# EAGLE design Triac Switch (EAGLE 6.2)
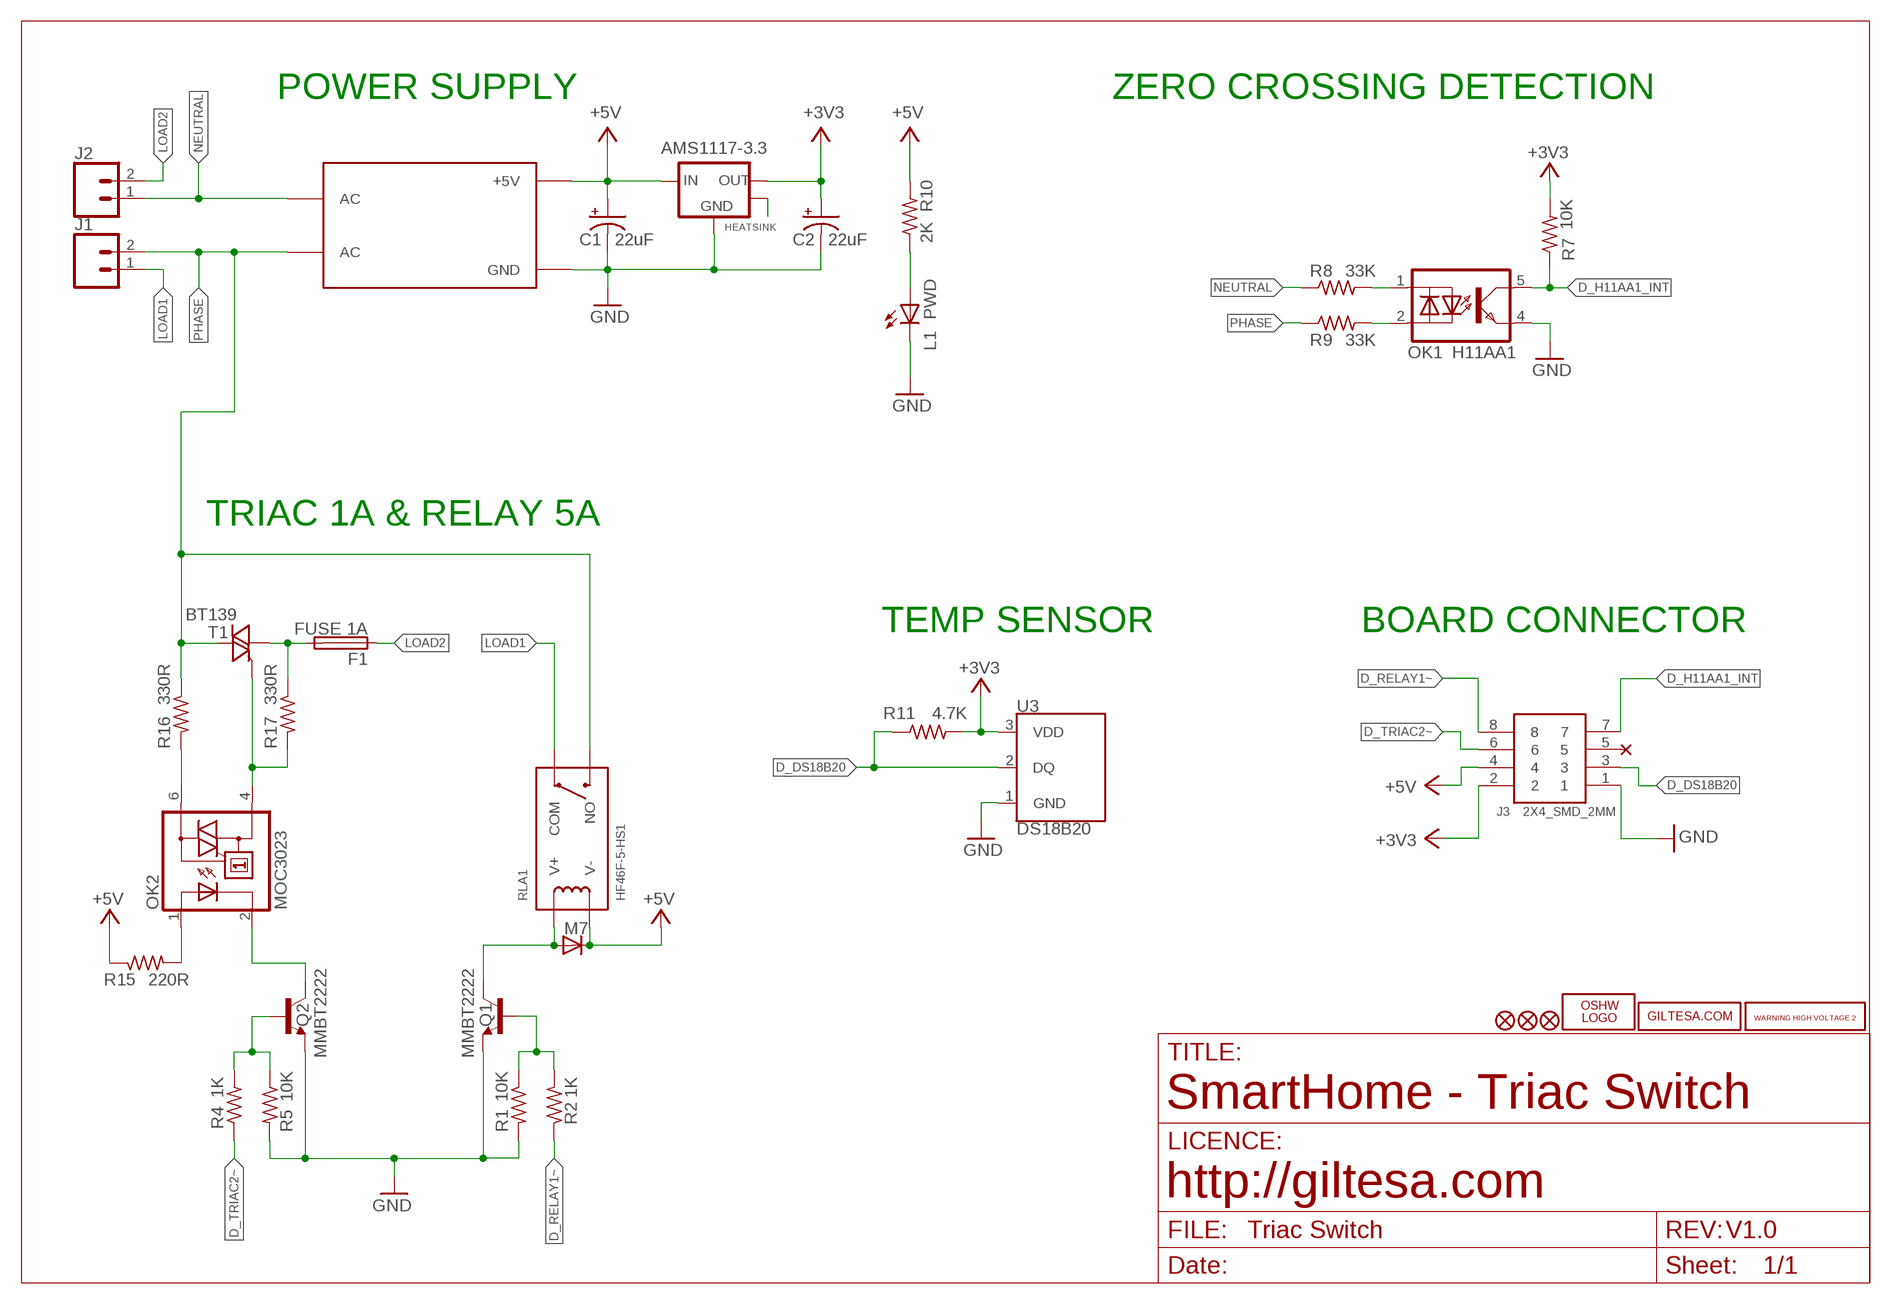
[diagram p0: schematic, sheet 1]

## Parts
AMS1117-3.3  AMS1117SOT89_2  [SOT89_2]
C1  22uF  CAP_POL3528  [EIA3528]
C2  22uF  CAP_POL3528  [EIA3528]
D1  M7  DIODE-SMB  [SMB]
F1  FUSE 1A  FUSETE5  [TE5]
J1  TERMINAL_5MM_2P_90º  [TERMINAL_5MM_2P_90º]
J2  TERMINAL_5MM_2P_90º  [TERMINAL_5MM_2P_90º]
J3  2X4_SMD_2MM  2X4_SMD_2.0MM  [2X4_SMD_2.0MM]
L1  PWD  LEDCHIP-LED0805  [CHIP-LED0805]
LOGO1  OSHW_LOGO_FILLX0150-NT  [OSHW_FILLX150_NOTEXT]
OK1  H11AA1  [H11AA1]
OK2  MOC3023  MOC3021MSMD  [DIL6-SMD]
Q1  MMBT2222  TRANSISTOR_NPNSOT23  [SOT23]
Q2  MMBT2222  TRANSISTOR_NPNSOT23  [SOT23]
R1  10K  R0603  [R0603]
R2  1K  R0603  [R0603]
R4  1K  R0603  [R0603]
R5  10K  R0603  [R0603]
R7  10K  R0603  [R0603]
R8  33K  R1206  [R1206]
R9  33K  R1206  [R1206]
R10  2K  R0603  [R0603]
R11  4.7K  R0603  [R0603]
R15  220R  R0603  [R0603]
R16  330R  R1206  [R1206]
R17  330R  R1206  [R1206]
RLA1  HF46F-5-HS1  RELAY_HF46F-5-HS1  [RELAY_HF46F-5-HS1]
T1  BT139  BT138-V  [TO220BV]
U3  DS18B20  [DS18B20]
U$1  HILINK_HLK-PM01_5V  [HILINK_HLK-PM01_5V]
U$4  WARNING_HIGH_VOLTAGE_2  [WARNING_HIGH_VOLTAGE_2]
U$5  GILTESA.COM_MASK  [GILTESA.COM_MASK]
U$6  FIDUCIAL1X2  [FIDUCIAL-1X2]
U$7  FIDUCIAL1X2  [FIDUCIAL-1X2]
U$14  FIDUCIAL1X2  [FIDUCIAL-1X2]

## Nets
+3V3: AMS1117-3.3.2(OUT) C2.A(+) J3.2 R7.2 R11.2 U3.3(VDD)
+5V: AMS1117-3.3.3(IN) C1.A(+) D1.C J3.4 R10.2 R15.1 RLA1.V- U$1.+5V
D_DS18B20: J3.3 R11.1 U3.2(DQ)
D_H11AA1_INT: J3.7 OK1.5 R7.1
D_RELAY1~: J3.8 R2.1
D_TRIAC2~: J3.6 R4.1
GND: AMS1117-3.3.1(GND) C1.C(-) C2.C(-) J3.1 L1.C OK1.4 Q1.2(E) Q2.2(E) R1.2 R5.2 U3.1(GND) U$1.GND
HEATSINK: AMS1117-3.3.4(NC)
LOAD1: J1.1 RLA1.COM
LOAD2: F1.1 J2.2
N$1: F1.2 R17.1 T1.T1(A1)
N$2: Q1.1(B) R1.1 R2.2
N$3: D1.A Q1.3(C) RLA1.V+
N$6: OK1.1 R8.2
N$7: OK1.2 R9.2
N$8: L1.A R10.1
N$10: OK2.1(A) R15.2
N$12: OK2.6(A2) R16.2
N$13: OK2.4(A1) R17.2 T1.G
N$46: Q2.1(B) R4.2 R5.1
N$47: OK2.2(C) Q2.3(C)
NEUTRAL: J2.1 R8.1 U$1.AC@2(AC)
PHASE: J1.2 R9.1 R16.1 RLA1.NO T1.T2(A2) U$1.AC@1(AC)
Unconnected: J3.5

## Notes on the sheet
- POWER SUPPLY | ZERO CROSSING DETECTION
- TRIAC 1A & RELAY 5A
- TEMP SENSOR | BOARD CONNECTOR
- SmartHome - Triac Switch
- http://giltesa.com
- V1.0

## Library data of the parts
AMS1117-3.3 = ,giltesa:AMS1117
C1 C2 = SparkFun:CAP_POL: Capacitor Polarized
D1 = diode:DIODE-: DIODE
F1 = fuse:FUSE: Fuse; OC_FARNELL: unknown; OC_NEWARK: unknown
J1 J2 = ,giltesa:TERMINAL_5MM_2P_90º
J3 = ,giltesa:2X4_SMD_2.0MM
L1 = led:LED: LED
LOGO1 = ohw-logo:OSHW_LOGO_FILL
OK1 = ,giltesa:H11AA1
OK2 = optocoupler:MOC30*M: RANDOM-PHASE OPTOISOLATORS TRIAC DRIVER OUTPUT Source: http://www.fairchildsemi.com MOC3020-M.pdf
Q1 Q2 = SparkFun:TRANSISTOR_NPN: Transistor NPN BJT configuration in SOT23 package. MMBT2222 is the common NPN we use. Double check BCE configuration again layout.
R1 R2 R4 R5 R7 R10 R11 R15 = ,giltesa:R0603
R8 R9 R16 R17 = ,giltesa:R1206
RLA1 = ,giltesa:RELAY_HF46F-5-HS1
T1 = triac:BT138: TRIAC Source: http://www.semiconductors.philips.com BT138_SERIES_2.pdf
U3 = ,giltesa:DS18B20
U$1 = ,giltesa:HILINK_HLK-PM01_5V
U$4 = ,giltesa_logos:WARNING_HIGH_VOLTAGE_2
U$5 = ,giltesa_logos:GILTESA.COM_MASK
U$6 U$7 U$14 = SparkFun:FIDUCIAL: Fiducial Alignment Points

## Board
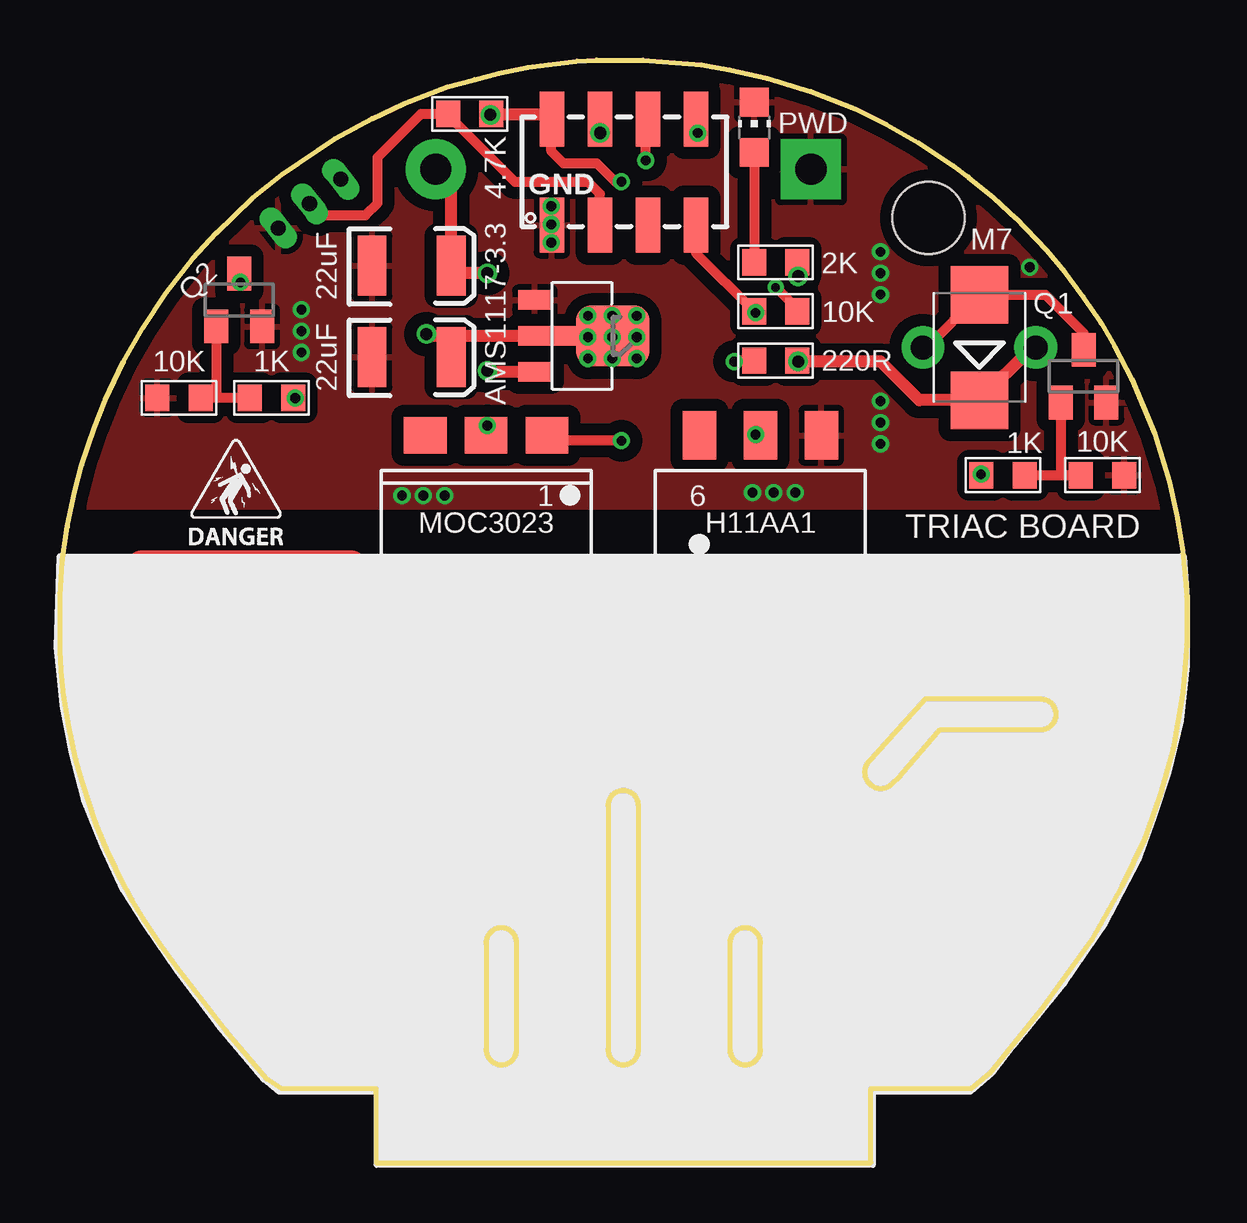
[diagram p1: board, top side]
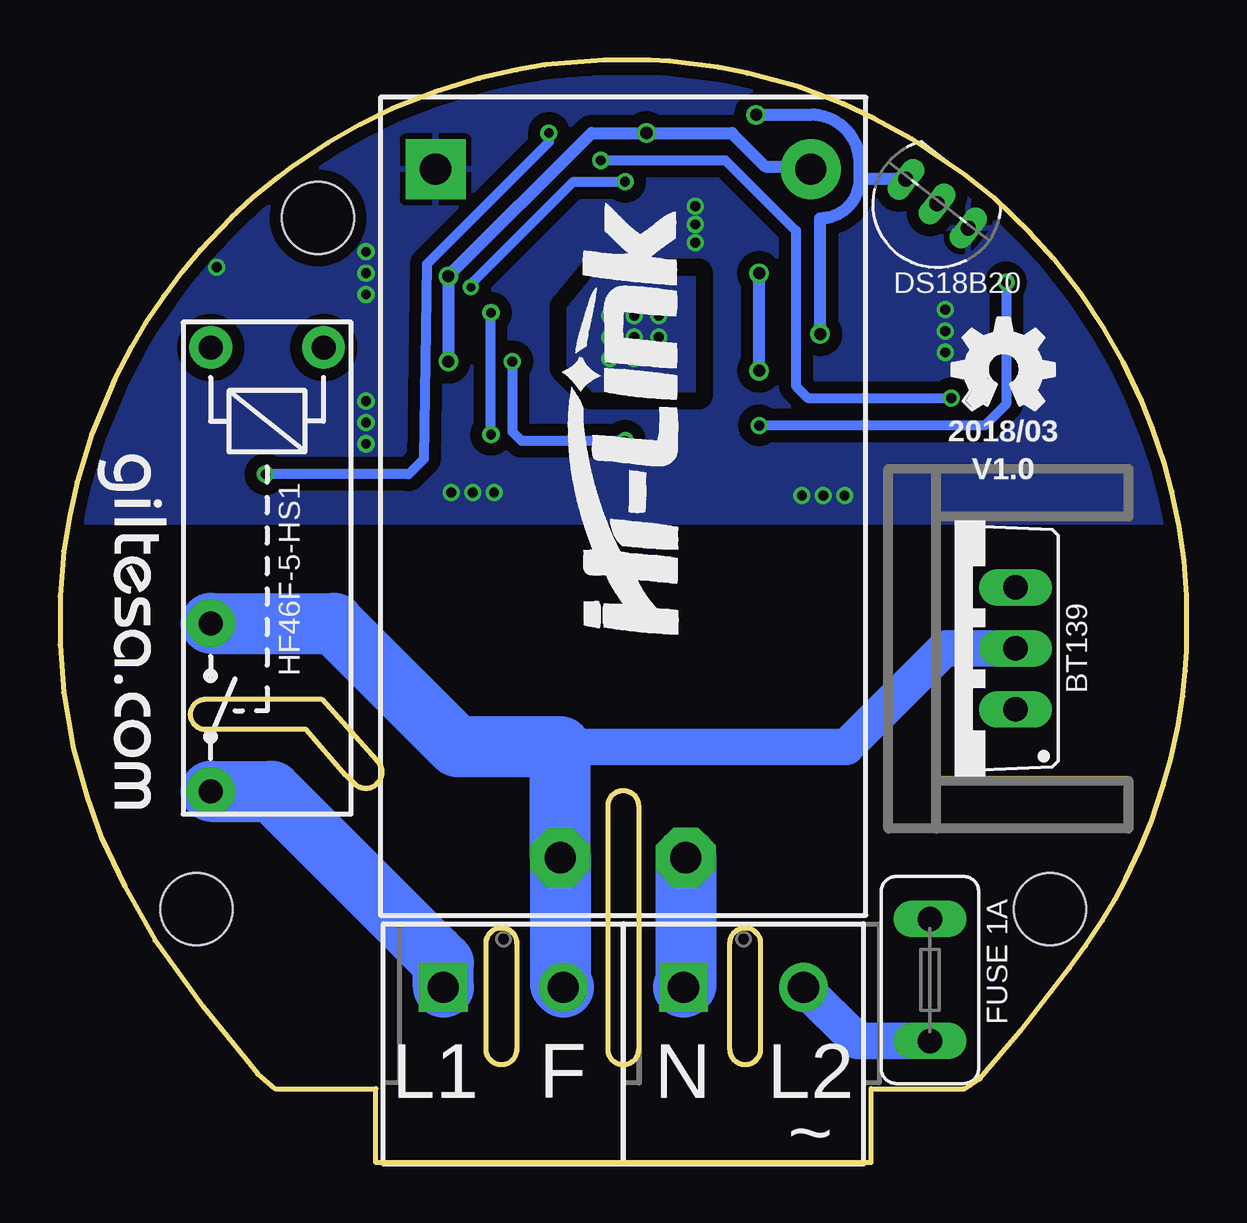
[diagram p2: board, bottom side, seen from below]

Size 46.94 x 45.97 mm. Coordinates in mm from the lower left corner, seen from the top.
Outline: 96 segments
Copper layers (1*16): Top 0.035mm / dielectric 1.6mm / Bottom 0.035mm
Design rules: minimum track width 6mil, minimum drill 12mil, track to track 6mil, track to pad 6mil, pad to pad 6mil, via to via 8mil, smd to smd 0mil, copper to edge 20mil, drill to drill 10mil, minimum pad ring 6mil, minimum via ring 6mil, stop-mask expansion 0mil, vias tented up to drill 100mil, thermal gap 10mil
Holes 3 mm at 5.69,10.57 41.25,10.57 36.19,39.38
bRestrict: 6 lines

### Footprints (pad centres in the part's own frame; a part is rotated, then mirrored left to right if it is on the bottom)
SOT89_2 = smd 0.8 x 1.4: 1 -1.499,-1.981; 3 1.499,-1.981 | smd 0.8 x 2.54: 2 0,-1.409 | smd 2.54 x 3.048: 4 0,1.27
EIA3528 = smd 1.2 x 2.5: A 1.65,0; C -1.65,0
SMB = smd 2.4 x 2.4: A 2.2,0; C -2.2,0
TE5 = drill 1.016 long: 1 -2.54,0; 2 2.54,0
TERMINAL_5MM_2P_90º = drill 1.3 pad 2.032 square: 1 0.004,0 | drill 1.3 pad 2.032: 2 5.004,0
2X4_SMD_2.0MM = smd 2.286 x 1.016: 1 -2.213,2.976; 2 2.212,2.976; 3 -2.213,0.976; 4 2.212,0.976; 5 -2.213,-1.024; 6 2.212,-1.024; 7 -2.213,-3.024; 8 2.212,-3.024
CHIP-LED0805 = smd 1.2 x 1.2: A 0,-1.05; C 0,1.05
H11AA1 = smd 1.397 x 2.032: 1 -2.54,-4.645; 2 0,-4.645; 3 2.54,-4.645; 4 2.54,4.645; 5 0,4.645; 6 -2.54,4.645
DIL6-SMD = smd 1.78 x 1.52: 1 -2.54,-4.645; 2 0,-4.645; 3 2.54,-4.645; 4 2.54,4.645; 5 0,4.645; 6 -2.54,4.645
SOT23 = smd 1 x 1.4: 1 -0.95,-1.1; 2 0.95,-1.1; 3 0,1.1
R0603 = smd 1 x 1.1: 1 -0.901,0.013; 2 0.901,0.013
R1206 = smd 1.6 x 1.8: 1 -1.387,-0.013; 2 1.362,-0.013
RELAY_HF46F-5-HS1 = drill 1 pad 2.032: COM 9.3,-2.35; NO 2.3,-2.35 | drill 1 pad 1.778: V+ -9.2,2.35; V- -9.2,-2.35
TO220BV = drill 1.016 long: G 2.54,-2.54; T1 -2.54,-2.54; T2 0,-2.54
DS18B20 = drill 0.635 pad 0.864 long: 1 -1.651,0; 2 0,0; 3 1.651,0
HILINK_HLK-PM01_5V = drill 1.3 pad 2.5: +5V 31.109,2.3 | drill 1.3 pad 2.5 octagon: AC@1 2.409,12.73; AC@2 2.409,7.5 | drill 1.3 pad 2.5 square: GND 31.109,17.93
FIDUCIAL-1X2 = smd 1 x 1: 1 0,0

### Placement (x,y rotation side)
AMS1117-3.3  21.76,34.46 270 top
C1  14.65,37.38 0 top
C2  14.65,33.57 0 top
D1  38.3,33.98 90 top
F1  10.69,7.62 90 bottom
J1  30.97,7.31 0 bottom
J2  20.97,7.31 0 bottom
J3  23.47,41.29 90 top
L1  28.93,43.16 0 top
LOGO1  9.75,31.39 0 bottom
OK1  29.18,25.67 0 top
OK2  17.75,25.67 180 top
Q1  42.65,32.78 0 top
Q2  7.47,35.96 0 top
R1  43.44,28.65 0 top
R2  39.29,28.65 0 top
R4  8.81,31.89 180 top
R5  4.96,31.89 180 top
R7  29.82,35.48 0 top
R8  24.92,17.39 0 top
R9  30.58,16 90 top
R10  29.82,37.51 0 top
R11  17.07,43.7 0 top
R15  29.82,33.45 180 top
R16  16.66,17.39 0 top
R17  2.44,21.44 90 top
RLA1  38.3,24.78 270 bottom
T1  9.66,21.44 90 bottom
U3  10.4,39.98 142 bottom
U$1  13.36,10.3 90 bottom
U$2  [ELECTROCUTION_SMALL]  5.14,25.63 0 top
U$4  43.03,15.51 0 top
U$5  45.44,29.61 270 bottom
U$6  32.42,1.37 90 top
U$7  23.47,24.66 90 top
U$14  14.54,1.37 90 top

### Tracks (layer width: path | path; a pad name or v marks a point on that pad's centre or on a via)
+3V3  (via drill 0.36, 0.41, 0.51)
  Top 0.406: R7.2 30.72,35.59 v29.82,36.5 | v23.39,40.89 23.14,40.89 22.38,41.65 20.98,41.65 20.47,42.16 20.47,43.48 J3.2
  Top 0.508: AMS1117-3.3.2 16.46,34.46 | 16.46,34.46 16.28,34.29 16.28,33.6 C2.A | 16.46,34.46 15.34,34.46 v15.27,34.54 | J3.2 20.28,43.71 R11.2 17.96,43.71 v17.93,43.68
  Bottom 0.406: v23.39,40.89 25.55,40.89 29.82,36.62 v29.82,36.5
  Bottom 0.508: v15.27,34.54 15.27,39.37 arc-90 13.61,41.02 | v17.93,43.68 15.65,43.68 arc90 13.61,41.65 13.61,41.02 | U3.3 13.59,40.99 arc90 13.61,41.02
+5V  (via drill 0.51)
  Top 0.508: RLA1.V- 40.51,33.98 D1.C 35.81,31.78 34.19,33.4 v30.76,33.4 R15.1 30.76,33.47 v30.76,33.4 | U$1.+5V 16.3,40.77 C1.A 16.61,37.08 v17.81,37.08 | J3.4 22.49,43.06 v22.5,42.92 | 30.82,37.52 R10.2 30.76,37.49 v30.76,36.95 | AMS1117-3.3.3 17.86,32.96 v17.81,33.02
  Bottom 0.508: v17.81,33.02 v17.81,37.08 | 15.66,41.38 U$1.+5V 15.77,41.52 17.55,41.52 18.95,42.92 v22.5,42.92 24.79,42.92 v30.76,36.95 v30.76,33.4
D_DS18B20
  Top 0.406: U3.2 10.4,39.92 10.82,39.49 12.73,39.49 13.23,40 13.23,41.91 15.04,43.71 R11.1 16.17,43.66 18.95,40.89 22,40.89 22.49,40.39 J3.3
D_H11AA1_INT  (via drill 0.41)
  Top 0.406: J3.7 26.49,37.92 R7.1 28.85,35.43 v28.98,35.43 | OK1.5 29.06,30.3 v28.98,30.35
  Bottom 0.406: v28.98,30.35 v28.98,35.43
D_RELAY1~  (via drill 0.41)
  Top 0.406: J3.8 26.49,43 v26.57,42.92 | v38.38,28.7 38.35,28.7 R2.1
  Bottom 0.406: v26.57,42.92 26.57,42.54 31.65,37.46 31.78,29.33 32.41,28.7 v38.38,28.7
D_TRIAC2~  (via drill 0.41)
  Top 0.406: v9.8,31.87 9.72,31.87 R4.1 | v24.41,41.78 24.41,43.42 J3.6
  Bottom 0.406: v9.8,31.87 15.77,31.87 16.28,32.38 16.28,38.86 19.2,41.78 v24.41,41.78
GND  (via drill 0.41)
  other vias: 20.47,39.87 20.47,39.11 20.47,38.35 40.41,37.33 34.19,29.97 34.19,30.86 34.19,31.75 30.63,27.94 29.74,27.94 28.85,27.94 14.25,27.81 15.14,27.81 16.03,27.81 10.06,35.56 10.06,34.67 10.06,33.78 34.19,37.97 34.19,37.08 34.19,36.19
  pour Top (isolate 0.508): -0.03,27.32 46.96,27.32 46.96,27.58 46.33,28.85 45.06,32.02 42.52,36.47 39.98,39.64 35.53,42.82 29.82,45.36 24.74,45.99 20.93,45.99 15.85,44.72 10.77,42.18 6.96,39.01 3.78,35.2 1.88,32.02 -0.03,27.58
  pour Bottom (isolate 0.508): -0.03,26.69 46.96,26.69 46.33,28.85 45.06,32.02 42.52,36.47 39.98,39.64 35.53,42.82 29.82,45.36 24.74,45.99 20.93,45.99 15.85,44.72 10.77,42.18 6.96,39.01 3.78,35.2 1.88,32.02
HEATSINK  (via drill 0.41)
  Top 0.406: AMS1117-3.3.4 22.25,34.46 v22,35.3
  other vias: 23.01,35.3 24.03,35.3 22,34.41 23.01,34.41 24.03,34.41 24.03,33.52 23.01,33.52 22,33.52
  pour Bottom: 20.47,32 20.47,36.95 24.79,36.95 25.81,35.68 25.81,33.14 24.79,32
LOAD1
  Bottom 2.54: RLA1.COM 38.12,15.48 31.33,8.7 31.01,8.38 30.97,8.33 J1.1
LOAD2
  Bottom 1.524: F1.1 13.73,5.08 J2.2
N$1
  Top 1.524: F1.2 10.69,16 8.53,18.16 7.26,18.16 | 7.26,18.16 3.45,18.16 2.44,19.17 2.44,20.04 R17.1 | T1.T1 7.12,18.3 7.26,18.16
N$2
  Top 0.406: R2.2 41.68,28.66 | 41.68,28.66 R1.1 | Q1.1 41.7,28.67 41.68,28.66
N$3
  Top 0.406: RLA1.V+ 36.11,33.98 D1.A 41.06,36.18 42.65,34.59 Q1.3
N$6
  Top 1.143: R8.2 26.28,20.66 OK1.1
N$7
  Top 1.143: OK1.2 29.18,19.6 30.63,18.16 30.63,17.4 R9.2
N$8
  Top 0.406: L1.A 28.93,37.54 R10.1
N$10  (via drill 0.41)
  Top 0.406: R15.2 28.13,33.43 v28.09,33.4 | v23.39,30.09 20.33,30.09 OK2.1
  Bottom 0.406: v28.09,33.4 28.09,30.48 27.71,30.09 v23.39,30.09
N$12
  Top 1.524: OK2.6 20.29,18.87 18.69,17.27 18.58,17.51 R16.2
N$13
  Top 1.524: 7.26,24.76 12.09,24.76 12.87,23.98 12.89,23.98 12.89,23.96 15.14,21.71 15.14,21.1 OK2.4 | 7.26,24.76 3.45,24.76 2.44,23.74 2.44,22.82 R17.2 | T1.G 7.12,24.62 7.26,24.76
N$46
  Top 0.406: R4.2 6.38,31.88 | 6.38,31.88 R5.1 | Q2.1 6.52,32.02 6.38,31.88
N$47  (via drill 0.41)
  Top 0.406: Q2.3 7.47,36.75 v7.52,36.7 | v17.81,30.73 17.34,30.73 OK2.2
  Bottom 0.406: v7.52,36.7 7.52,31.62 8.41,30.73 v17.81,30.73
NEUTRAL
  Top 1.143: U$1.AC@2 20.86,14.71 R8.1
  Bottom 2.54: U$1.AC@2 20.86,7.41 J2.1
PHASE
  Top 1.143: R9.1 30.59,14.05 29.62,13.08 29.36,12.82 29.25,12.71 U$1.AC@1
  Top 1.524: T1.T2 10.07,21.44 14.12,17.39 15.26,17.39 R16.1
  Bottom 1.524: 26.09,17.34 14.18,17.34 10.07,21.44 T1.T2
  Bottom 2.54: RLA1.NO 35.53,22.48 30.38,17.34 26.09,17.34 U$1.AC@1 26.09,7.44 J1.2

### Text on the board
tPlace: GND | 1 | 6 | TRIAC BOARD
bPlace: 2018/03 | V1.0 | L2 | N | F | L1 | ~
